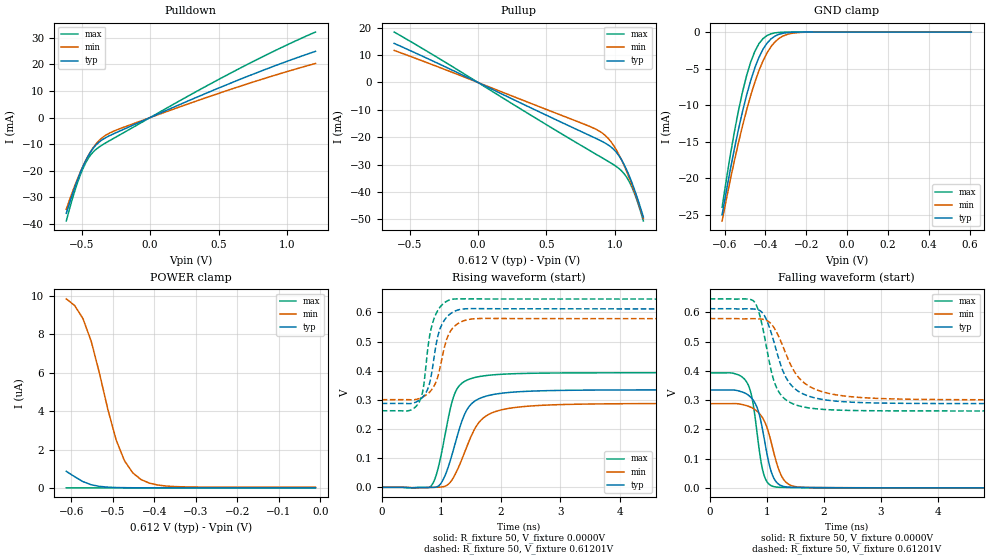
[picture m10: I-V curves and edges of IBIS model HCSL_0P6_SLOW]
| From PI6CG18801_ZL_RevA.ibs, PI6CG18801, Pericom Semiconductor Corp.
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[Model]   HCSL_0P6_SLOW
Model_type Output
Vref=0.6000V
Vmeas=900mV
| variable   typ   min   max
C_comp   2.000pF   1.970pF   2.030pF
[Voltage Range]   0.61201V   0.57834V   0.64563V
[POWER Clamp Reference]   0.61201V   0.57834V   0.64563V
[GND Clamp Reference]   0.0000V   0.0000V   0.0000V
[Pullup Reference]   0.61201V   0.57834V   0.64563V
[Pulldown Reference]   0.0000V   0.0000V   0.0000V
[Temperature Range]   25   85   -40
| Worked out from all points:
|   slope of the pulldown table from 0 to 0.092 V, typ, clamps not added: 43.8 ohm
|   slope of the pullup table from 0 to 0.092 V, typ, clamps not added: 41.4 ohm
|   GND clamp passes 1 mA (typ) near -0.37 V on its own axis
|   falling waveform, R_fixture 50, V_fixture 0.0000V: 20-80 % time 218ps typ, 268ps min, 175ps max; typ from 0.334 V to 0 V
|   rising waveform, R_fixture 50, V_fixture 0.0000V: 20-80 % time 323ps typ, 401ps min, 250ps max; typ from 0 V to 0.334 V
|   falling waveform, R_fixture 50, V_fixture 0.61201V: 20-80 % time 372ps typ, 478ps min, 276ps max; typ from 0.612 V to 0.288 V
|   rising waveform, R_fixture 50, V_fixture 0.61201V: 20-80 % time 189ps typ, 220ps min, 166ps max; typ from 0.288 V to 0.612 V
[GND Clamp]
| Voltage   I(typ)   I(min)   I(max)
-612mV    -25.02mA   -25.88mA   -24mA
-572mV    -18.86mA   -20.25mA   -16.88mA
-552mV    -16mA      -17.64mA   -13.68mA
-512mV    -10.87mA   -12.84mA   -8.188mA
-492mV    -8.627mA   -10.67mA   -5.955mA
-452mV    -4.921mA   -6.891mA   -2.659mA
-432mV    -3.494mA   -5.314mA   -1.606mA
-392mV    -1.518mA   -2.854mA   -474.6uA
-372mV    -924.8uA   -1.975mA   -235.2uA
-332mV    -299.3uA   -841.7uA   -49.75uA
-252mV    -21.66uA   -107.3uA   -1.344uA
608mV     1.088nA    32.69nA    -5.916pA
[POWER Clamp]
| Voltage   I(typ)   I(min)   I(max)
-612mV    861nA      9.857uA    1.622nA
-592mV    584.2nA    9.512uA    621.3pA
-572mV    326.3nA    8.835uA    247.2pA
-552mV    161.3nA    7.648uA    107.3pA
-512mV    36.25nA    4.099uA    34.37pA
-492mV    17.5nA     2.503uA    26.17pA
-472mV    8.826nA    1.419uA    22.47pA
-452mV    4.814nA    782.1nA    20.43pA
-432mV    2.956nA    432.9nA    19.01pA
-392mV    1.685nA    147.6nA    16.72pA
-352mV    1.395nA    67.95nA    14.59pA
-12.01mV  1.099nA    32.4nA     -3.301pA
[Pulldown]
| Voltage   I(typ)   I(min)   I(max)
-612mV    -36.03mA   -34.49mA   -38.92mA
-572mV    -29.56mA   -28.64mA   -31.37mA
-532mV    -23.7mA    -23.29mA   -24.78mA
-492mV    -18.59mA   -18.51mA   -19.38mA
-472mV    -16.38mA   -16.35mA   -17.2mA
-432mV    -12.73mA   -12.62mA   -13.91mA
-392mV    -10.14mA   -9.725mA   -11.83mA
-312mV    -7.227mA   -6.264mA   -9.161mA
27.99mV   641.2uA    526.5uA    828.2uA
568mV     12.54mA    10.27mA    16.19mA
908mV     19.41mA    15.88mA    25.08mA
1.208V    24.93mA    20.36mA    32.2mA
[Pullup]
| Voltage   I(typ)   I(min)   I(max)
-612mV    14.27mA    11.7mA     18.42mA
-272mV    6.49mA     5.323mA    8.39mA
768mV     -18.25mA   -15.07mA   -23.43mA
908mV     -21.57mA   -18.47mA   -27.55mA
968mV     -23.42mA   -21.41mA   -29.33mA
1.008V    -25.33mA   -24.4mA    -30.61mA
1.048V    -28.19mA   -28.22mA   -32.24mA
1.088V    -32.14mA   -32.77mA   -34.75mA
1.108V    -34.49mA   -35.27mA   -36.51mA
1.148V    -39.84mA   -40.66mA   -41.16mA
1.168V    -42.79mA   -43.54mA   -44.01mA
1.208V    -49.14mA   -49.69mA   -50.59mA
[Falling Waveform]
R_fixture = 50
V_fixture = 0.0000V
V_fixture_min = 0.0000V
V_fixture_max = 0.0000V
|   Time   V(typ)   V(min)   V(max)
0s        334.3mV    287.6mV    392.9mV
420ps     334.3mV    287.8mV    391.1mV
660ps     319.1mV    279.9mV    357.6mV
750ps     302.9mV    272.5mV    299.6mV
855ps     260.2mV    257.2mV    149.6mV
930ps     195.4mV    238.2mV    59.41mV
1.095ns   45.81mV    142.4mV    5.945mV
1.275ns   6.023mV    34.89mV    1.574mV
1.5ns     1.45mV     4.207mV    1.006mV
5ns       22.99uV    33.46uV    17.95uV
[Rising Waveform]
R_fixture = 50
V_fixture = 0.0000V
V_fixture_min = 0.0000V
V_fixture_max = 0.0000V
|   Time   V(typ)   V(min)   V(max)
0s        8.328uV    9.007uV    8.298uV
820ps     -121.4uV   -261.1uV   2.946mV
920ps     1.306mV    180uV      45.89mV
1.02ns    22.41mV    1.633mV    134.7mV
1.24ns    155.8mV    47.53mV    328.4mV
1.42ns    262.6mV    135.2mV    366.5mV
1.62ns    302.6mV    219.3mV    379.2mV
2ns       322.3mV    265.2mV    387.6mV
2.8ns     331.6mV    282.3mV    391.8mV
10ns      334.3mV    287.6mV    392.9mV
[Falling Waveform]
R_fixture = 50
V_fixture = 0.61201V
V_fixture_min = 0.57834V
V_fixture_max = 0.64563V
|   Time   V(typ)   V(min)   V(max)
0s        612mV      578.3mV    645.6mV
780ps     610.9mV    577.9mV    636.2mV
880ps     605.6mV    577.1mV    587.6mV
980ps     580.6mV    573.4mV    496.6mV
1.18ns    461.3mV    528.6mV    339mV
1.36ns    369mV      446.4mV    297.3mV
1.64ns    320.7mV    361.1mV    276.5mV
2.1ns     298.6mV    322.1mV    266.8mV
3ns       289.7mV    305.1mV    263.3mV
10ns      287.7mV    300.6mV    262.7mV
[Rising Waveform]
R_fixture = 50
V_fixture = 0.61201V
V_fixture_min = 0.57834V
V_fixture_max = 0.64563V
|   Time   V(typ)   V(min)   V(max)
0s        287.7mV    300.6mV    262.7mV
445ps     287mV      300.6mV    262.6mV
625ps     298.3mV    304.2mV    291.2mV
700ps     312.1mV    310.9mV    343.3mV
790ps     348.1mV    324.1mV    501.9mV
850ps     407mV      338.2mV    560.9mV
970ps     538.9mV    402.3mV    615.7mV
1.135ns   592.5mV    529.2mV    642.3mV
1.6ns     612.7mV    578.7mV    646mV
5ns       612mV      578.3mV    645.6mV
[Ramp]
| variable   typ   min   max
dV/dt_r   0.20059V/322.42p   0.17257V/400.25p   0.23564V/249.53p
dV/dt_f   0.19440V/371.76p   0.16661V/477.89p   0.22964V/275.53p
R_load = 50
